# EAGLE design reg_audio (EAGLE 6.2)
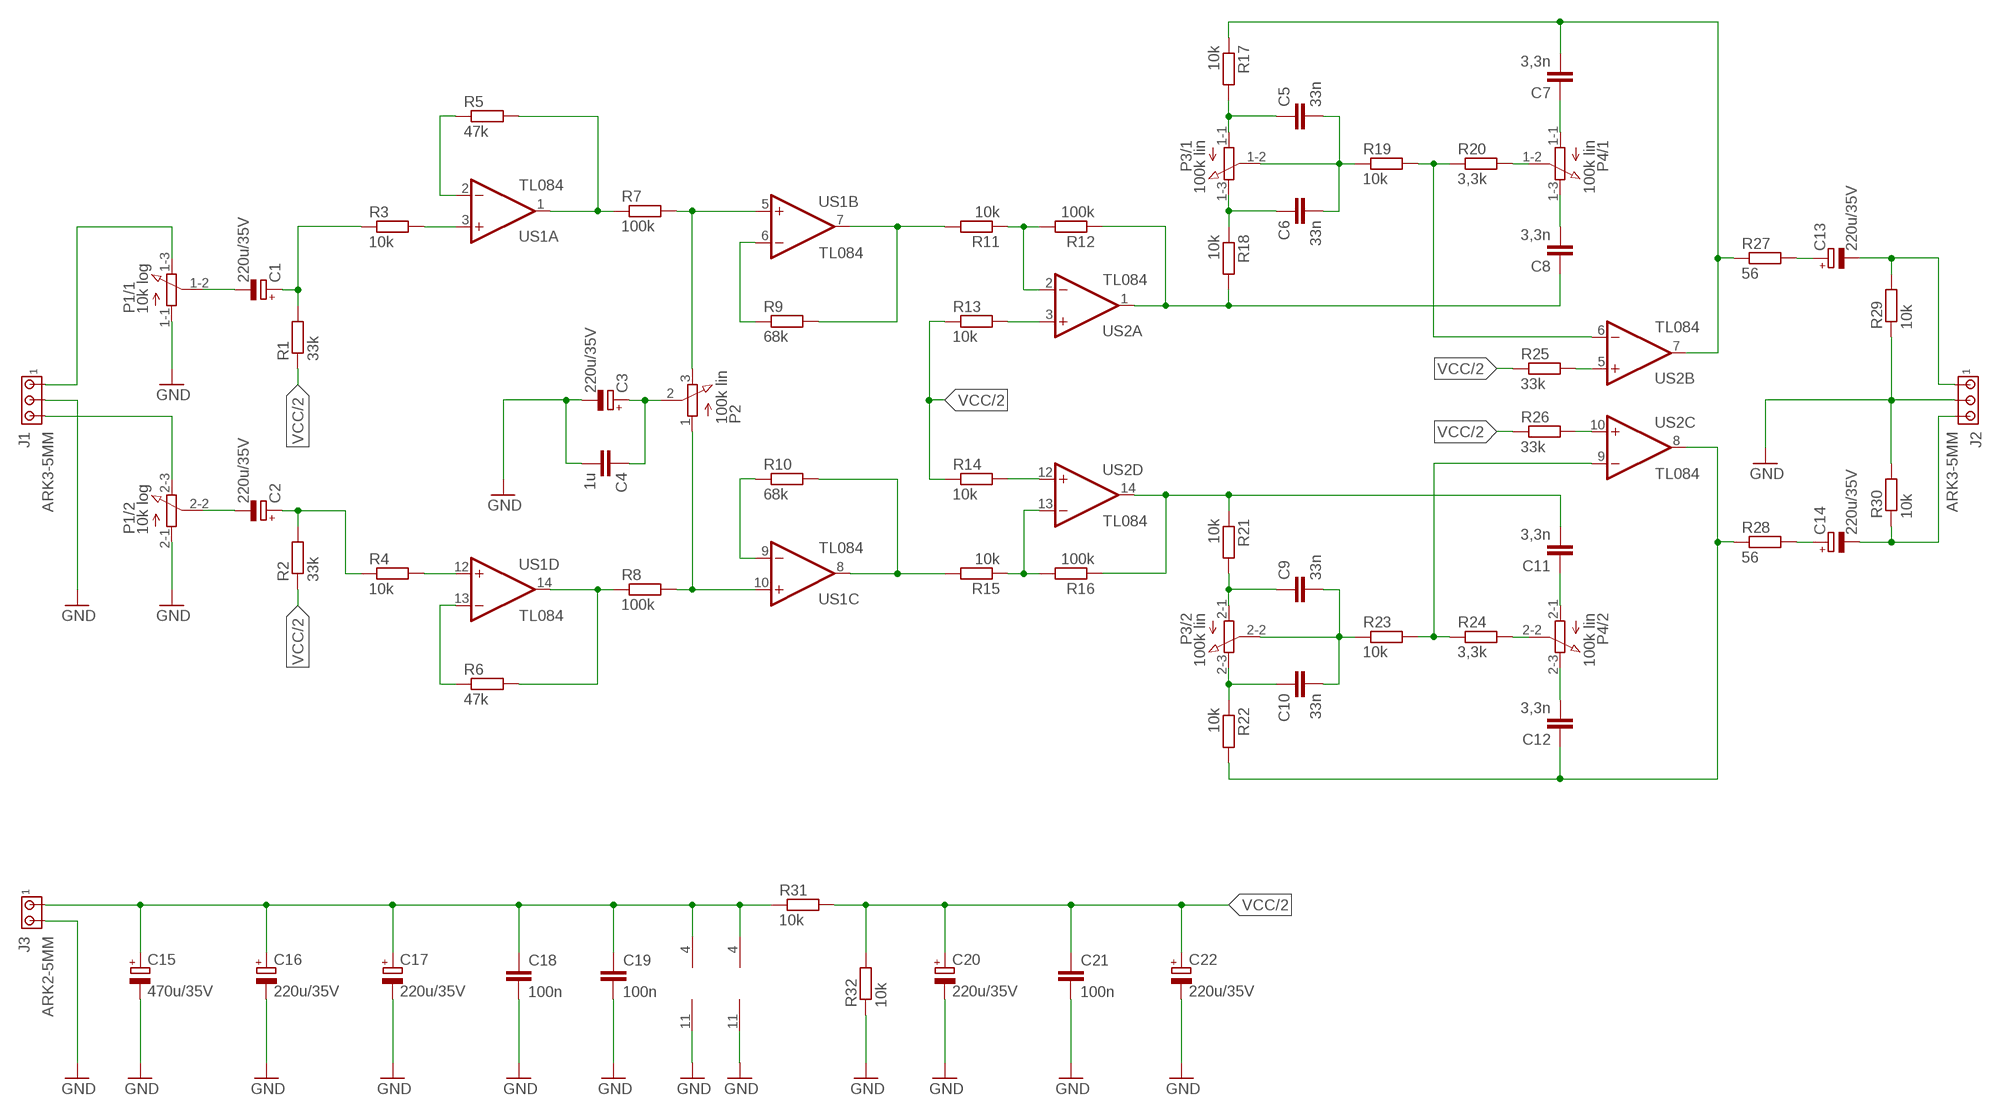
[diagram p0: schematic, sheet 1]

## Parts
C1  220u/35V  CPOL-EUE3.5-8  [E3,5-8]
C2  220u/35V  CPOL-EUE3.5-8  [E3,5-8]
C3  220u/35V  CPOL-EUE3.5-8  [E3,5-8]
C4  1u  C-EU050-050X075  [C050-050X075]
C5  33n  C-EU050-025X075  [C050-025X075]
C6  33n  C-EU050-025X075  [C050-025X075]
C7  3,3n  C-EU050-025X075  [C050-025X075]
C8  3,3n  C-EU050-025X075  [C050-025X075]
C9  33n  C-EU050-025X075  [C050-025X075]
C10  33n  C-EU050-025X075  [C050-025X075]
C11  3,3n  C-EU050-025X075  [C050-025X075]
C12  3,3n  C-EU050-025X075  [C050-025X075]
C13  220u/35V  CPOL-EUE3.5-8  [E3,5-8]
C14  220u/35V  CPOL-EUE3.5-8  [E3,5-8]
C15  470u/35V  CPOL-EUE5-10.5  [E5-10,5]
C16  220u/35V  CPOL-EUE3.5-8  [E3,5-8]
C17  220u/35V  CPOL-EUE3.5-8  [E3,5-8]
C18  100n  C-EU050-025X075  [C050-025X075]
C19  100n  C-EU050-025X075  [C050-025X075]
C20  220u/35V  CPOL-EUE3.5-8  [E3,5-8]
C21  100n  C-EU050-025X075  [C050-025X075]
C22  220u/35V  CPOL-EUE3.5-8  [E3,5-8]
J1  ARK3-5MM  [3PIN-5MM]
J2  ARK3-5MM  [3PIN-5MM]
J3  ARK2-5MM  [2PIN-5MM]
P1  10k log  3RP/1610G  [POT_PODWOJNY]
P2  100k lin  3RP/1610N  [POT_POJEDYNCZY]
P3  100k lin  3RP/1610G  [POT_PODWOJNY]
P4  100k lin  3RP/1610G  [POT_PODWOJNY]
R1  33k  R-EU_0207/7  [0207/7]
R2  33k  R-EU_0207/7  [0207/7]
R3  10k  R-EU_0207/7  [0207/7]
R4  10k  R-EU_0207/7  [0207/7]
R5  47k  R-EU_0207/7  [0207/7]
R6  47k  R-EU_0207/7  [0207/7]
R7  100k  R-EU_0207/7  [0207/7]
R8  100k  R-EU_0207/7  [0207/7]
R9  68k  R-EU_0207/7  [0207/7]
R10  68k  R-EU_0207/7  [0207/7]
R11  10k  R-EU_0207/7  [0207/7]
R12  100k  R-EU_0207/7  [0207/7]
R13  10k  R-EU_0207/7  [0207/7]
R14  10k  R-EU_0207/7  [0207/7]
R15  10k  R-EU_0207/7  [0207/7]
R16  100k  R-EU_0207/7  [0207/7]
R17  10k  R-EU_0207/7  [0207/7]
R18  10k  R-EU_0207/7  [0207/7]
R19  10k  R-EU_0207/7  [0207/7]
R20  3,3k  R-EU_0207/7  [0207/7]
R21  10k  R-EU_0207/7  [0207/7]
R22  10k  R-EU_0207/7  [0207/7]
R23  10k  R-EU_0207/7  [0207/7]
R24  3,3k  R-EU_0207/7  [0207/7]
R25  33k  R-EU_0207/7  [0207/7]
R26  33k  R-EU_0207/7  [0207/7]
R27  56  R-EU_0207/7  [0207/7]
R28  56  R-EU_0207/7  [0207/7]
R29  10k  R-EU_0207/7  [0207/7]
R30  10k  R-EU_0207/7  [0207/7]
R31  10k  R-EU_0207/7  [0207/7]
R32  10k  R-EU_0207/7  [0207/7]
US1  TL084  TL084P  [DIL14]
US2  TL084  TL084P  [DIL14]

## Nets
GND: C3.- C4.2 C15.- C16.- C17.- C18.2 C19.2 C20.- C21.2 C22.- J1.P$2 J2.P$2 J3.P$2 P1.1-1(/1:A) P1.2-1(/2:A) R29.1 R30.2 R32.1 US1.11(P:V-) US2.11(P:V-)
LL: R10.2 R15.2 US1.8(C:OUT)
N$1: J1.P$1 P1.1-3(/1:E)
N$2: J1.P$3 P1.2-3(/2:E)
N$3: C1.- P1.1-2(/1:S)
N$4: C2.- P1.2-2(/2:S)
N$5: R11.1 R12.2 US2.2(A:-IN)
N$6: C8.1 R12.1 R18.2 US2.1(A:OUT)
N$7: R15.1 R16.2 US2.13(D:-IN)
N$8: C11.2 R16.1 R21.1 US2.14(D:OUT)
N$9: C6.1 P3.1-3(/1:E) R18.1
N$10: C5.1 P3.1-1(/1:A) R17.2
N$11: C5.2 C6.2 P3.1-2(/1:S) R19.1
N$12: R19.2 R20.1 US2.6(B:-IN)
N$13: P4.1-2(/1:S) R20.2
N$14: C12.2 P4.2-3(/2:E)
N$15: C11.1 P4.2-1(/2:A)
N$16: C7.2 R17.1 R27.1 US2.7(B:OUT)
N$17: R25.2 US2.5(B:+IN)
N$18: C9.1 P3.2-1(/2:A) R21.2
N$19: C10.1 P3.2-3(/2:E) R22.1
N$20: C9.2 C10.2 P3.2-2(/2:S) R23.1
N$21: C12.1 R22.2 R28.1 US2.8(C:OUT)
N$22: R23.2 R24.1 US2.9(C:-IN)
N$23: P4.2-2(/2:S) R24.2
N$24: C8.2 P4.1-3(/1:E)
N$25: C7.1 P4.1-1(/1:A)
N$26: R26.2 US2.10(C:+IN)
N$27: R13.2 US2.3(A:+IN)
N$28: R14.2 US2.12(D:+IN)
N$29: R9.2 R11.2 US1.7(B:OUT)
N$31: R9.1 US1.6(B:-IN)
N$32: R10.1 US1.9(C:-IN)
N$33: P2.1(A) R8.2 US1.10(C:+IN)
N$34: P2.3(E) R7.2 US1.5(B:+IN)
N$35: C1.+ R1.2 R3.1
N$36: C2.+ R2.2 R4.1
N$37: R6.1 US1.13(D:-IN)
N$38: R6.2 R8.1 US1.14(D:OUT)
N$39: R5.2 R7.1 US1.1(A:OUT)
N$40: R5.1 US1.2(A:-IN)
N$41: R3.2 US1.3(A:+IN)
N$42: R4.2 US1.12(D:+IN)
N$43: C13.+ R27.2
N$44: C13.- J2.P$1 R29.2
N$45: C14.+ R28.2
N$46: C14.- J2.P$3 R30.1
N$47: C15.+ C16.+ C17.+ C18.1 C19.1 J3.P$1 R31.1 US1.4(P:V+) US2.4(P:V+)
N$48: C3.+ C4.1 P2.2(S)
VCC/2: C20.+ C21.1 C22.+ R1.1 R2.1 R13.1 R14.1 R25.1 R26.1 R31.2 R32.2

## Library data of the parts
C1-C3 C13-C17 C20 C22 = rcl:CPOL-EU: POLARIZED CAPACITOR, European symbol
C4-C12 C18 C19 C21 = rcl:C-EU: CAPACITOR, European symbol
J1 J2 = zlacza_futrzak:ARK3: ARK 3 Raster 5mm i 3,5mm
J3 = zlacza_futrzak:ARK2: ARK 2
P1 P3 P4 = inne_futrzak:3RP/1610G: 16mm Potentiometer two level Source: http://www.alphapotentiometers.net/html/16mm_pot_2.html
P2 = inne_futrzak:3RP/1610N: 16mm Potentiometer one level Source: http://www.alphapotentiometers.net/html/16mm_pot_2.html
R1-R32 = rcl:R-EU_: RESISTOR, European symbol
US1 US2 = linear:TL084: OP AMP

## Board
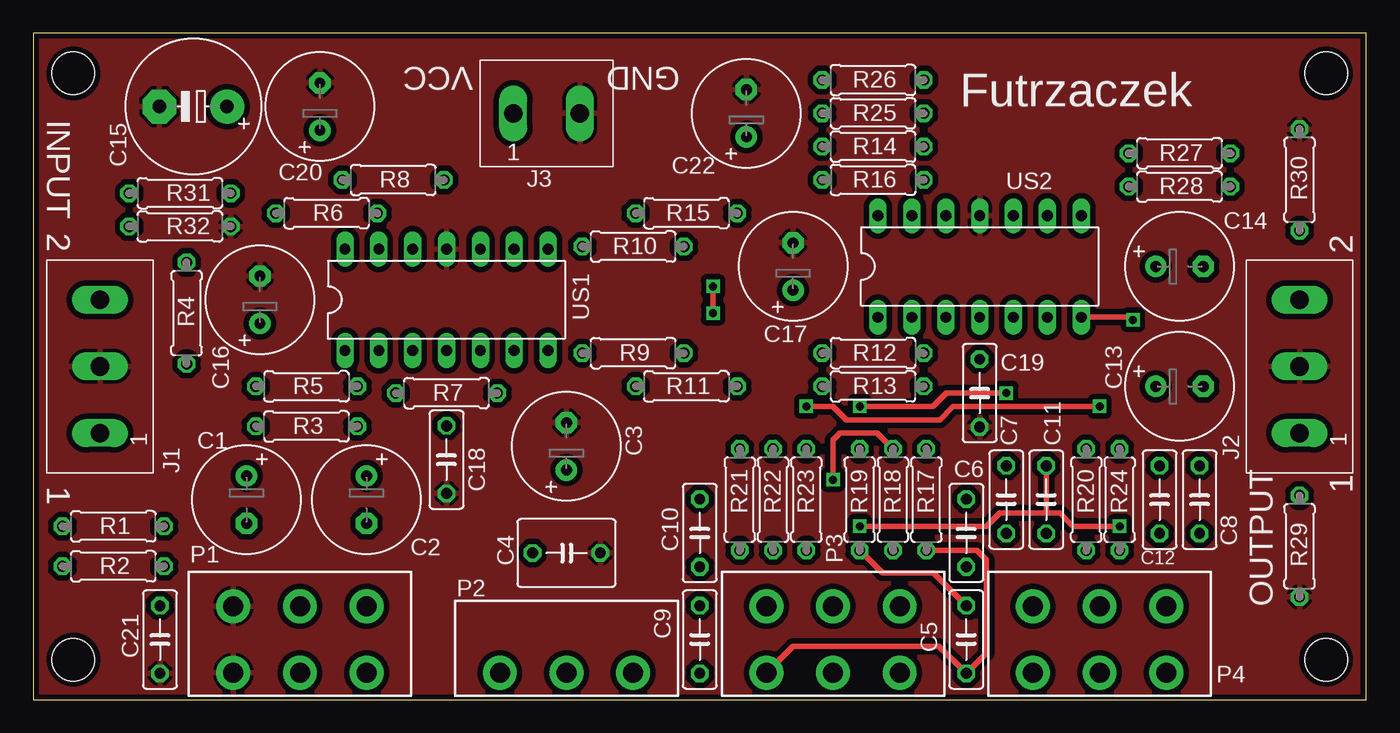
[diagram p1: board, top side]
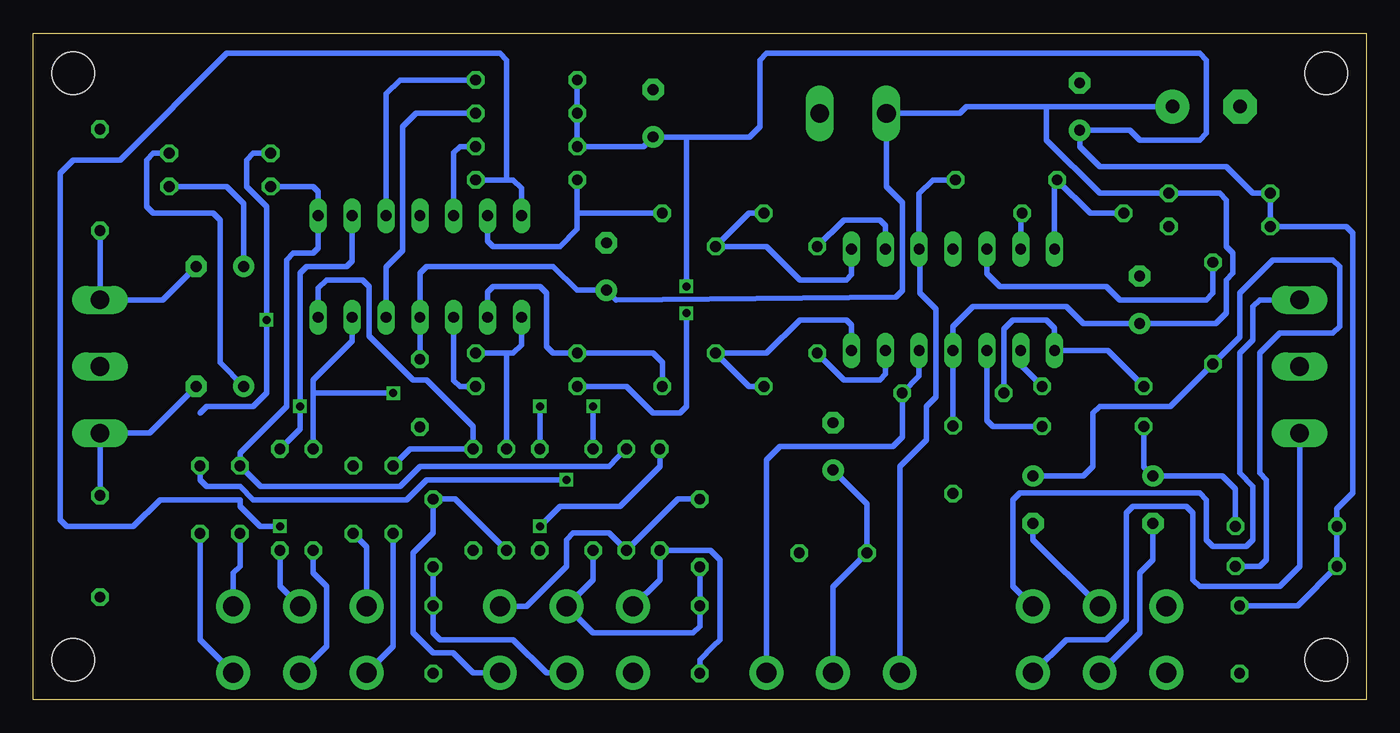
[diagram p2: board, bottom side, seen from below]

Size 100 x 50 mm. Coordinates in mm from the lower left corner, seen from the top.
Outline: 0,0 100,0 100,50 0,50 0,0
Copper layers (1*16): Top 0.035mm / dielectric 1.5mm / Bottom 0.035mm
Design rules: minimum track width 10mil, minimum drill 23mil, track to track 8mil, track to pad 8mil, pad to pad 8mil, via to via 8mil, smd to smd 8mil, copper to edge 15mil, drill to drill 8mil, minimum pad ring 10mil, minimum via ring 8mil, stop-mask expansion 4mil, vias tented up to drill 0mil, thermal gap 10mil
Holes 3.2 mm at 3,3 97,3 3,47 97,47

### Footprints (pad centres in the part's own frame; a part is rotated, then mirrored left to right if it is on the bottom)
E3,5-8 = drill 0.813 pad 1.6: + -1.778,0 | drill 0.813 pad 1.6 octagon: - 1.778,0
C050-050X075 = drill 0.813 octagon: 1 -2.54,0; 2 2.54,0
C050-025X075 = drill 0.813 octagon: 1 -2.54,0; 2 2.54,0
E5-10,5 = drill 1.016 pad 2.54: + -2.54,0 | drill 1.016 pad 2.54 octagon: - 2.54,0
3PIN-5MM = drill 1.4 long: P$1 -5,0; P$2 0,0; P$3 5,0
2PIN-5MM = drill 1.4 long: P$1 -2.5,0; P$2 2.5,0
POT_PODWOJNY = drill 1.5 pad 2.54: 1-1 -5,0; 1-2 0,0; 1-3 5,0; 2-1 -5,5; 2-2 0,5; 2-3 5,5
POT_POJEDYNCZY = drill 1.5 pad 2.54: 1 -5,0; 2 0,0; 3 5,0
0207/7 = drill 0.813 octagon: 1 -3.81,0; 2 3.81,0
DIL14 = drill 0.813 long: 1 -7.62,-3.81; 2 -5.08,-3.81; 3 -2.54,-3.81; 4 0,-3.81; 5 2.54,-3.81; 6 5.08,-3.81; 7 7.62,-3.81; 8 7.62,3.81; 9 5.08,3.81; 10 2.54,3.81; 11 0,3.81; 12 -2.54,3.81; 13 -5.08,3.81; 14 -7.62,3.81

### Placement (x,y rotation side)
C1  16,15 270 top
C2  25,15 270 top
C3  40,19 90 top
C4  40,11 0 top
C5  70,4.5 90 top
C6  70,12.5 270 top
C7  73,15 90 top
C8  87.5,15 270 top
C9  50,4.5 90 top
C10  50,12.5 270 top
C11  76,15 90 top
C12  84.5,15 270 top
C13  86,23.5 0 top
C14  86,32.5 0 top
C15  12,44.5 180 top
C16  17,30 90 top
C17  57,32.5 90 top
C18  31,18 270 top
C19  71,23 270 top
C20  21.5,44.5 90 top
C21  9.5,4.5 270 top
C22  53.5,44 90 top
J1  5,25 90 top
J2  95,25 90 top
J3  38.5,44 0 top
P1  20,2 0 top
P2  40,2 0 top
P3  60,2 0 top
P4  80,2 0 top
R1  6,13 0 top
R2  6,10 0 top
R3  20.5,20.5 0 top
R4  11.5,29 90 top
R5  20.5,23.5 180 top
R6  22,36.5 180 top
R7  31,23 0 top
R8  27,39 0 top
R9  45,26 0 top
R10  45,34 0 top
R11  49,23.5 180 top
R12  63,26 180 top
R13  63,23.5 0 top
R14  63,41.5 0 top
R15  49,36.5 180 top
R16  63,39 180 top
R17  67,15 270 top
R18  64.5,15 90 top
R19  62,15 90 top
R20  79,15 270 top
R21  53,15 270 top
R22  55.5,15 90 top
R23  58,15 90 top
R24  81.5,15 270 top
R25  63,44 0 top
R26  63,46.5 0 top
R27  86,41 0 top
R28  86,38.5 0 top
R29  95,11.5 90 top
R30  95,39 90 top
R31  11,38 180 top
R32  11,35.5 180 top
US1  31,30 0 top
US2  71,32.5 0 top

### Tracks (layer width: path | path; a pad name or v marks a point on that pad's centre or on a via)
GND
  pour Top (isolate 0.406): 0,0 100,0 100,50 0,50
LL
  Bottom 0.406: US1.8 38.62,31.88 39,31.5 42.5,31.5 45,34 R10.2 46.31,36.5 R15.2
N$1
  Bottom 0.406: J1.P$1 5,10 6.5,8.5 12.5,8.5 13,9 13,14 13.5,14.5 17.5,14.5 18,14 18,6 19.5,4.5 22.5,4.5 P1.1-3
N$2
  Bottom 0.406: J1.P$3 8,30 8.5,29.5 8.5,27 9.5,26 9.5,17 8.5,16 8.5,12 9,11.5 11.5,11.5 12,12 12,14 12,15 12.5,15.5 26,15.5 26.5,15 26.5,8.5 P1.2-3
N$3
  Bottom 0.406: C1.- 16,10.5 17,9.5 17,5 P1.1-2
N$4
  Bottom 0.406: C2.- 25,12 P1.2-2
N$5
  Bottom 0.406: US2.2 65.92,30.58 65.5,31 62,31 61.5,30.5 61.5,26.5 61,26 R12.2 53.5,26 52.81,25.31 R11.1
N$6  (via drill 0.6)
  Top 0.406: v60,16.5 60,19.5 60.5,20 63.31,20 R18.2
  Bottom 0.406: US2.1 63.38,26.62 64,26 64.5,26 | 64.5,26 R12.1 | R18.2 64.5,26 | C8.1 87.5,16.5 87,16 84.5,16 83.5,15 72.5,15 72,15 70.5,16.5 v60,16.5
N$7
  Bottom 0.406: R16.2 59.19,36.5 | 59.19,36.5 59.19,35.31 60.5,34 65.5,34 65.92,34.42 US2.13 | R15.1 59.19,36.5
N$8  (via drill 0.6)
  Top 0.406: v62,13 71.5,13 72.5,14 76,14 | 76,14 77,14 78,13 v81.5,13 | C11.2 76,14
  Bottom 0.406: US2.14 63.38,38.38 64,39 64.5,39 | 64.5,39 R16.1 | 64.5,39 64.5,48 65,48.5 85.5,48.5 93.5,40.5 97,40.5 98,39.5 98,13.5 97.5,13 92.5,13 90.5,15 84.5,15 84.5,14.5 83,13 v81.5,13 | R21.1 53,17.5 56,14.5 60.5,14.5 v62,13
N$9
  Bottom 0.406: R18.1 68.35,15.04 C6.1 70,12.5 71.5,11 71.5,10.5 71.5,5 71,4.5 70.5,4 70,3.5 68.5,3.5 67,2 P3.1-3
N$10
  Top 0.406: R17.2 70.81,11.19 71.5,10.5 71.5,3.46 C5.1 67.96,4 57,4 P3.1-1
N$11
  Top 0.406: C5.2 67.54,9.5 63.69,9.5 R19.1
  Bottom 0.406: C6.2 C5.2 70,5 69.5,4.5 64,4.5 61.5,2 P3.1-2
N$12  (via drill 0.6)
  Top 0.406: v62,22 67.5,22 68.5,23 v73,23
  Bottom 0.406: US2.6 76.08,26.92 79,24 79,23 | 79,23 R20.1 | R19.2 v62,22 | v73,23 79,23
N$13
  Bottom 0.406: R20.2 79,9.5 78,8.5 78,4 P4.1-2
N$14
  Bottom 0.406: P4.2-3 85,9.5 84.5,10 C12.2
N$15
  Bottom 0.406: P4.2-1 75,11.46 C11.1
N$16  (via drill 0.6)
  Top 0.406: US2.7 82.31,28.69 v82.5,28.5
  Bottom 0.406: R27.1 83.5,41 84,40.5 84,38.5 82.5,37 v82.5,28.5 82.5,23 83.5,22 87,22 87.5,21.5 | US2.7 78.62,30.88 78,31.5 75.3,31.5 74.8,31 74.8,27.3 71.5,24 70.5,24 67,20.5 R17.1 71.73,18.81 C7.2
N$17
  Bottom 0.406: US2.5 73.54,32.46 72.3,33.7 72.3,43 71.3,44 R25.2
N$18
  Bottom 0.406: C9.1 50,3 49,4 48.5,4.5 48.5,10.5 49,11 49.19,11.19 R21.2 53,9 P3.2-1
N$19
  Bottom 0.406: C10.1 51.65,15.04 R22.1 56.81,12.5 59.5,12.5 60,12 60,11.5 60,10 63,7 P3.2-3
N$20
  Bottom 0.406: C10.2 C9.2 50,5.5 50.5,5 58,5 P3.2-2 58,9 R23.1
N$21
  Bottom 0.406: R28.1 79,38.5 78.62,38.12 US2.8 78.62,33.88 79,33.5 80.5,33.5 81,33 81,22 83,20 84.5,18.5 C12.1 82.96,16 74.54,16 74.5,16 72.5,16 71,17.5 56.81,17.5 56.16,18.16 R22.2
N$22  (via drill 0.6)
  Top 0.406: v58,22 60,22 61,21 68,21 69,22 v80,22
  Bottom 0.406: US2.9 76.08,32.92 76.5,32.5 79.5,32.5 80,32 80,23.5 v80,22 80,20.31 R24.1 | R23.2 v58,22
N$23
  Bottom 0.406: R24.2 81.5,8.5 P4.2-2
N$24
  Bottom 0.406: C8.2 87.5,4.5 P4.1-3
N$25
  Bottom 0.406: C7.1 73,4 P4.1-1
N$26
  Bottom 0.406: US2.10 73.54,45.46 72.5,46.5 R26.2
N$27
  Bottom 0.406: US2.3 68.46,23.96 68,23.5 R13.2
N$28
  Bottom 0.406: US2.12 68.46,41.04 68,41.5 R14.2
N$29
  Bottom 0.406: US1.7 38.62,28.12 39,28.5 42.5,28.5 45,26 R9.2 46.31,23.5 R11.2
N$31
  Bottom 0.406: US1.6 36.08,24.42 36.5,24 39.19,24 R9.1
N$32
  Bottom 0.406: US1.9 36.08,35.58 36.5,36 39.19,36 R10.1
N$33
  Bottom 0.406: R8.2 32.5,39 33.54,37.96 US1.10 33.5,33.77 33.5,30.5 32.3,29.3 32.3,22.7 33,22 33,19.5 35,17.5 P2.1
N$34
  Bottom 0.406: US1.5 33.54,24.27 R7.2 34.81,19.69 35.5,19 44,19 45,18 P2.3
N$35
  Bottom 0.406: R3.1 16.69,17.47 C1.+ 13.59,16.78 10.78,16.78 10.5,16.5 9.81,15.81 R1.2
N$36
  Bottom 0.406: C2.+ 21.22,16.78 20.5,17.5 20.5,21.5 20,22 14.69,22 R4.1 9.5,27.19 9.5,30.5 7,33 2.5,33 2,32.5 2,28 2.5,27.5 6.5,27.5 8,26 8,17 7.5,16.5 7.5,10.5 8,10 R2.2
N$37
  Bottom 0.406: US1.13 25.92,36.39 R6.1
N$38
  Bottom 0.406: R6.2 20.69,36.5 R8.1 23.38,38.81 US1.14
N$39
  Bottom 0.406: R7.1 27.19,27.81 26.5,28.5 24,28.5 23.38,27.88 US1.1 19.38,26.19 R5.2
N$40
  Bottom 0.406: US1.2 25.92,25.11 R5.1
N$41
  Bottom 0.406: US1.3 28.46,20.96 28,20.5 R3.2
N$42
  Bottom 0.406: US1.12 28.46,31.96 27.5,31 19.5,31 18.5,30 12,30 11.5,30.5 R4.2
N$43
  Bottom 0.406: R27.2 91,41 91.5,40.5 91.5,37 91,36.5 86.5,36.5 86,36 86,25.28 C13.+
N$44
  Bottom 0.406: C13.- 91.28,20 J2.P$1 R29.2
N$45
  Bottom 0.406: C14.+ 84.22,37.22 85.5,38.5 R28.2
N$46
  Bottom 0.406: C14.- 90.28,30 J2.P$3 R30.1
N$47
  Bottom 0.406: 24,44.5 30,44.5 30.5,44 J3.P$1 36,38.5 34.8,37.3 34.8,30.7 35.3,30.2 56.28,30 C17.+ 59.22,30.72 61,32.5 70.5,32.5 71,32 US2.4 C19.1 | 24,44.5 C15.+ | C18.1 US1.4 31,28 29.5,29.5 22.5,29.5 21.22,28.22 C16.+ 11.28,28.22 10.5,29 10.5,31.5 10,32 10,33.5 10.5,34 10.5,37.5 11,38 R31.1 20,38 24,42 24,44.5
N$48
  Bottom 0.406: P2.2 40,8.46 C4.1 37.46,13.92 37.46,14.68 C3.+
VCC/2  (via drill 0.6)
  Top 0.406: v51,29 v51,31
  Bottom 0.406: C21.1 5.15,7.04 R2.1 R1.1 2.19,14.31 1,15.5 1,35 1.5,35.5 R32.2 R31.2 8.5,38 10.5,40 20,40 21.5,41.5 C20.+ 17.72,42.72 17,42 12.5,42 12,42.5 12,48 12.5,48.5 45,48.5 45.5,48 45.5,43 46.28,42.22 51,42.22 | R26.1 R25.1 R14.1 54.22,41.5 C22.+ 51,42.22 | R13.1 55.5,23.5 53.5,21.5 51.5,21.5 51,22 v51,29 | v51,31 51,42.22

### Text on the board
tPlace: VCC | GND | INPUT | Futrzaczek | 2 | 2 | 1 | 1 | OUTPUT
